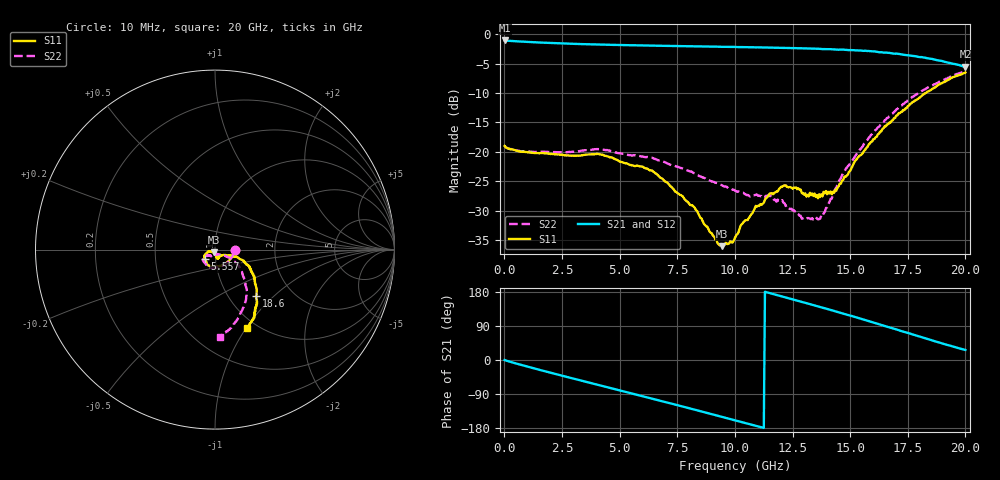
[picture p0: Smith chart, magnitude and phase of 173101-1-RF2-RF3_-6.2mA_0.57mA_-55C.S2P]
!  2-Port S-parameters saved by WinCal
! VAR MeasName=S-Parameters (CALIBRATED_DATA) read from VNA (N5242A)
! VAR MeasDate=2017-7-20 10:24:46
! VAR NAME=173101-1-RF2-RF3_-6.2mA_0.57mA_-55C
! VAR FILENAME=173101-1-RF2-RF3_-6.2mA_0.57mA_-55C.S2P
! VAR DATE=2017-7-20 10:24:46
! VAR PHYS_PORTS=1,2
# Hz S DB R 50
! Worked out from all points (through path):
!   401 points, 10 MHz to 20 GHz, reference 50 ohm
!   highest |S21| = -1.08 dB at 10 MHz (marker M1); lowest = -5.5 dB at 20 GHz (marker M2)
!   group delay of S21, straight-line fit = 45.8 ps
!   lowest |S11| = -36.0 dB at 9.455 GHz (marker M3), VSWR 1.03, Z = 49.6 - j1.53 ohm
!   |S11| at or under -10 dB: start of sweep to 18.27 GHz
!   |S22| runs from -31.7 to -6.3 dB; largest |S21 - S12| = 0.0094
!   S11 on the Smith chart (normalised r, x): 10 MHz: 1.25, -0.01; 5.557 GHz: 0.89, -0.10; 18.6 GHz: 1.34, -0.78; 20 GHz: 0.90, -1.01
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1e7  -18.98 -2.5  -1.08 -0.1  -1.09 -0.1  -18.94 -2.4
1.559225e9  -20.22 -55.5  -1.43 -26.5  -1.45 -26.5  -19.99 -55.4
3.358325e9  -20.57 -99.0  -1.70 -54.8  -1.71 -54.8  -19.78 -96.4
4.157925e9  -20.41 -114.8  -1.78 -67.1  -1.80 -67.1  -19.53 -111.4
5.557225e9  -22.30 -136.0  -1.88 -88.8  -1.90 -88.8  -20.60 -127.6
6.70665e9  -24.15 -152.0  -1.97 -106.8  -1.97 -106.7  -21.45 -140.4
8.255875e9  -29.50 -164.0  -2.09 -131.0  -2.10 -131.0  -23.63 -148.9
9.255375e9  -35.53 -114.6  -2.13 -147.0  -2.14 -147.0  -25.32 -141.6
9.455275e9  -36.00 -103.6  -2.15 -150.1  -2.16 -150.2  -25.70 -142.4
1.0005e10  -34.56 -78.5  -2.18 -159.0  -2.21 -159.0  -26.57 -140.8
1.030485e10  -32.24 -73.9  -2.20 -163.8  -2.22 -163.9  -26.92 -135.5
1.090455e10  -29.16 -73.3  -2.25 -173.4  -2.27 -173.5  -27.28 -126.4
1.205398e10  -25.91 -75.7  -2.34 167.7  -2.36 167.7  -28.19 -117.9
1.290355e10  -27.03 -62.7  -2.41 153.4  -2.41 153.3  -31.35 -93.3
1.335332e10  -27.07 -63.5  -2.47 145.8  -2.44 145.7  -31.24 -75.3
1.375312e10  -27.20 -57.7  -2.53 138.9  -2.52 138.8  -30.75 -62.4
1.430285e10  -26.93 -42.8  -2.60 129.4  -2.62 129.4  -26.79 -41.1
1.530235e10  -21.13 -23.1  -2.75 111.8  -2.77 111.6  -20.18 -29.6
1.670165e10  -15.01 -22.2  -3.19 86.1  -3.27 85.7  -13.96 -40.7
1.76012e10  -11.88 -32.8  -3.64 69.7  -3.65 69.5  -10.93 -51.5
1.86007e10  -9.23 -48.2  -4.27 50.9  -4.33 50.9  -8.64 -65.9
2e10  -6.52 -67.5  -5.53 26.5  -5.59 27.1  -6.26 -86.9
